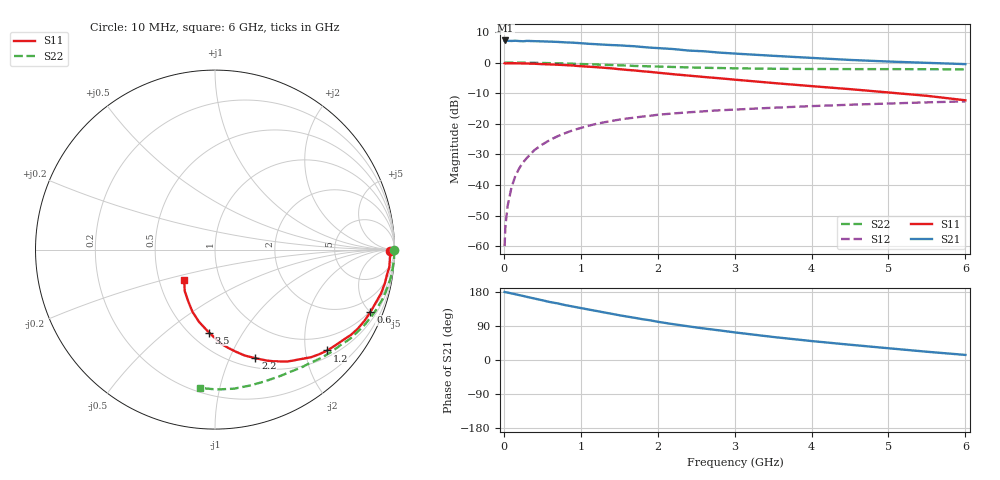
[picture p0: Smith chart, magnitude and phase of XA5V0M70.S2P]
! SIEMENS Discrete & RF Semiconductors
! BFY180
! Si NPN RF Bipolar Junction Transistor in MICRO-X
! VCE = 5 V  IC = 0.7 mA
! Common Emitter S-Parameters:  May  1997
# GHz  S  MA  R  50
!  f  S11  S21  S12  S22
! GHz  MAG  ANG  MAG  ANG  MAG  ANG  MAG  ANG
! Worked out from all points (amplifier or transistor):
!   36 points, 10 MHz to 6 GHz, reference 50 ohm
!   highest |S21| = 7.2 dB at 20 MHz (marker M1)
!   |S21| within 3 dB of that: start of sweep to 2.279 GHz
!   unconditionally stable (mu >= 1): 4.898 GHz to end of sweep
!   at 250 MHz: K = 0.05, MSG = 19.8 dB, |S12| = -32.6 dB
!   at 1.4 GHz: K = 0.43, MSG = 12.4 dB, |S12| = -19.1 dB
!   at 6 GHz: K = 1.03, MAG = 5.0 dB, |S12| = -12.7 dB
!   S11 on the Smith chart (normalised r, x): 10 MHz: 76, -22; 600 MHz: 0.93, -5.00; 1.2 GHz: 0.64, -2.47; 2.2 GHz: 0.60, -1.25; 3.5 GHz: 0.61, -0.72; 6 GHz: 0.67, -0.24
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0.01  0.9761 -0.4  2.255 179.5  0.001 85.0  0.999 -0.2
0.02  0.9652 -0.8  2.299 178.9  0.0021 82.6  0.9999 -0.5
0.05  0.9762 -1.6  2.268 177.9  0.0046 84.6  0.9984 -1.2
0.1  0.9757 -3.8  2.256 175.7  0.0092 88.1  0.9987 -2.4
0.15  0.976 -5.9  2.274 173.6  0.0141 86.6  0.9992 -3.6
0.2  0.9706 -7.4  2.247 171.2  0.0187 84.6  0.9957 -4.8
0.3  0.965 -11.1  2.262 166.6  0.0277 81.8  0.9932 -7.2
0.4  0.9572 -14.7  2.238 162.1  0.0374 79.8  0.9908 -9.6
0.6  0.933 -21.9  2.199 152.9  0.0544 74.0  0.9788 -14.2
0.8  0.9095 -29.0  2.139 144.7  0.0705 68.8  0.9639 -18.8
1.1  0.8571 -38.5  2.029 133.3  0.0926 61.3  0.939 -25.2
1.2  0.8412 -41.9  1.997 129.5  0.0995 58.6  0.931 -27.3
1.5  0.7803 -51.2  1.913 118.1  0.117 52.5  0.9033 -33.1
1.7  0.7434 -57.0  1.848 111.4  0.1261 48.9  0.8813 -36.6
2.2  0.6457 -69.6  1.665 94.6  0.1474 40.6  0.848 -44.9
2.6  0.5819 -78.3  1.531 83.2  0.1599 35.5  0.8226 -50.6
3  0.5263 -86.2  1.404 72.9  0.1705 30.8  0.806 -56.1
3.5  0.464 -94.1  1.291 60.8  0.1828 26.1  0.7926 -62.5
4  0.4122 -102.5  1.193 50.0  0.1944 21.3  0.7852 -68.9
4.5  0.3681 -110.0  1.105 40.3  0.2047 17.2  0.7821 -75.6
5.5  0.2863 -126.1  0.99 21.8  0.2238 8.8  0.7795 -89.3
6  0.2419 -135.2  0.944 13.4  0.2324 4.3  0.7752 -96.2
